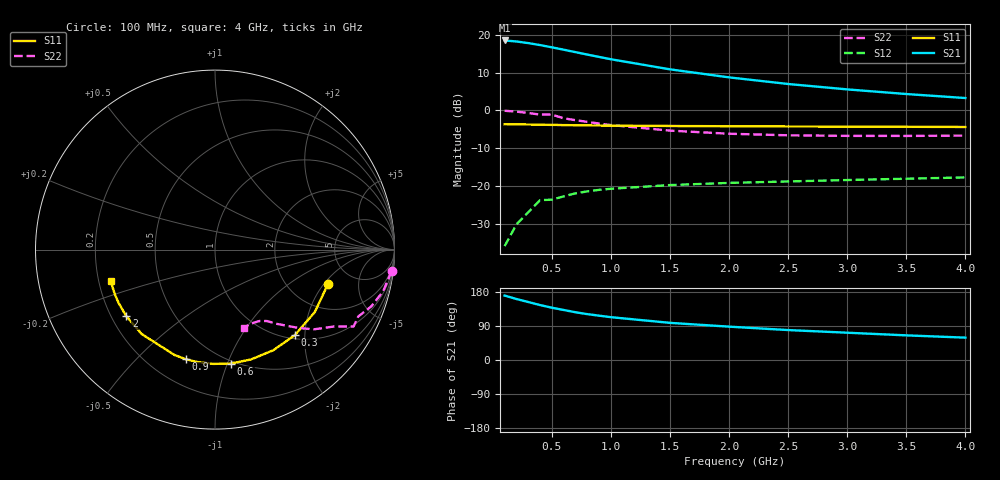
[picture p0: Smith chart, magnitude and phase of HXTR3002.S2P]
! HXTR-3002 Common Emitter
! Vce= 18v  Ic=30mA
# ghz s ma r 50
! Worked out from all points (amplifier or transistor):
!   16 points, 100 MHz to 4 GHz, reference 50 ohm
!   highest |S21| = 18.5 dB at 100 MHz (marker M1)
!   |S21| within 3 dB of that: start of sweep to 685.4 MHz
!   unconditionally stable (mu >= 1): 3.047 GHz to end of sweep
!   at 300 MHz: K = 0.11, MSG = 22.4 dB, |S12| = -26.9 dB
!   at 900 MHz: K = 0.35, MSG = 17.6 dB, |S12| = -21.0 dB
!   at 4 GHz: K = 1.19, MAG = 7.8 dB, |S12| = -17.7 dB
!   S11 on the Smith chart (normalised r, x): 100 MHz: 3.25, -2.21; 300 MHz: 1.07, -1.78; 600 MHz: 0.48, -1.03; 900 MHz: 0.35, -0.71; 2 GHz: 0.26, -0.31; 4 GHz: 0.25, -0.14
0.1  0.658 -17.0  8.44 170.0  0.016 82.0  0.991 -7.0
0.2  0.656 -32.0  8.18 161.0  0.031 75.0  0.965 -14.0
0.3  0.652 -47.0  7.79 153.0  0.045 68.0  0.926 -20.0
0.4  0.648 -60.0  7.33 145.0  0.065 62.0  0.881 -25.0
0.5  0.644 -72.0  6.85 138.0  0.066 56.0  0.883 -29.0
0.6  0.641 -82.0  6.37 132.0  0.073 52.0  0.787 -33.0
0.7  0.637 -91.0  5.91 126.0  0.08 48.0  0.744 -36.0
0.8  0.634 -99.0  5.49 121.0  0.085 45.0  0.706 -39.0
0.9  0.632 -105.0  5.11 117.0  0.089 42.0  0.671 -41.0
1  0.629 -111.0  4.76 113.0  0.092 39.0  0.641 -43.0
1.5  0.623 -131.0  3.5 98.0  0.103 32.0  0.541 -50.0
2  0.618 -143.0  2.74 88.0  0.11 29.0  0.492 -54.0
2.5  0.614 -151.0  2.24 79.0  0.115 28.0  0.469 -58.0
3  0.611 -156.0  1.9 72.0  0.12 27.0  0.461 -62.0
3.5  0.608 -160.0  1.65 65.0  0.125 27.0  0.46 -66.0
4  0.604 -163.0  1.46 59.0  0.13 27.0  0.465 -70.0
